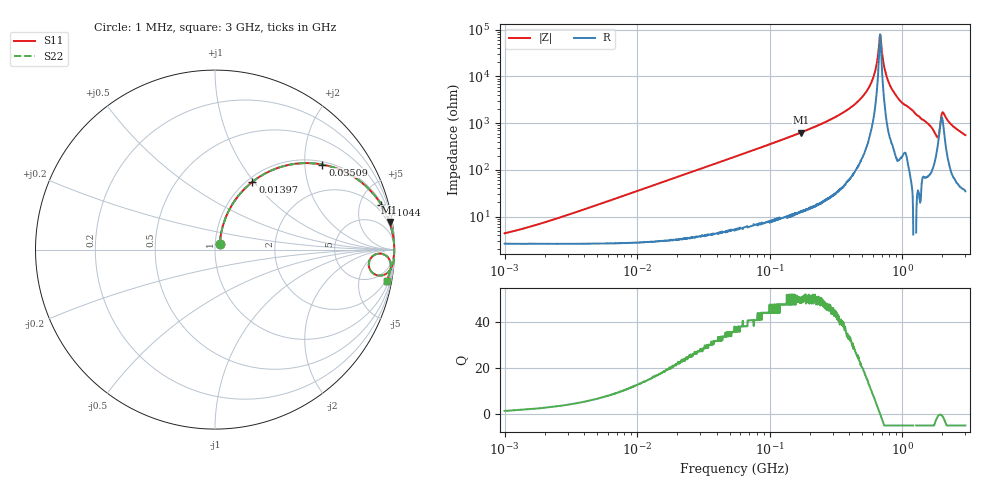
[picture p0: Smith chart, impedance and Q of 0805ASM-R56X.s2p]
!s-Parameter Generated by FASTRON Sdn. Bhd.
!FASTRON P/N : 0805ASM-R56X
!Keysight Technologies: E4991B_MY54100416_A.01.15
!Date: Fri Jun 19 14:53:02 2026
!Version  :Rev00  Fri Jun 19 14:53:02 2026
!Data & Calibration Information:
!Freq  S11  S21  S12  S22
!PortZ  Port1:50+j0  Port2:50+j0
!When reading reference impedance value at option line is always used.
! Remarks : This data is being provided solely for informational purposes.
# Hz S dB R 50
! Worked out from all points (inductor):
!   1601 points, 1 MHz to 3 GHz, reference 50 ohm
!   read as one part in series: L = 560 nH near 2.216 MHz
!   highest Q = 51.2 at 172.3 MHz (marker M1), where L = 581 nH
!   self-resonance near 682.1 MHz
!   S11 on the Smith chart (normalised r, x): 1 MHz: 1.05, +0.07; 13.97 MHz: 1.06, +0.98; 35.09 MHz: 1.08, +2.45; 104.4 MHz: 1.16, +7.37; 3 GHz: 2, -11
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1000000  -27.40 51.3  -0.23 -2.0  -0.23 -2.0  -27.40 51.3
3804036  -17.60 71.5  -0.30 -7.4  -0.30 -7.4  -17.60 71.5
1.397259e7  -7.31 61.1  -1.14 -25.5  -1.14 -25.5  -7.31 61.1
1.447069e7  -7.07 60.4  -1.20 -26.3  -1.20 -26.3  -7.07 60.4
3.508696e7  -2.35 38.4  -4.13 -49.7  -4.13 -49.7  -2.35 38.4
5.504702e7  -1.13 27.1  -6.82 -61.3  -6.82 -61.3  -1.13 27.1
1.044488e8  -0.36 15.1  -11.70 -73.7  -11.70 -73.7  -0.36 15.1
1.722755e8  -0.13 9.0  -16.10 -79.9  -16.10 -79.9  -0.13 9.0
2.083556e8  -0.09 7.2  -18.00 -81.6  -18.00 -81.6  -0.09 7.2
3.649251e8  -0.03 3.3  -24.80 -85.2  -24.80 -85.2  -0.03 3.3
5.077325e8  -0.01 1.5  -31.70 -85.6  -31.70 -85.6  -0.01 1.5
6.049187e8  -0.01 0.6  -39.50 -82.4  -39.50 -82.4  -0.01 0.6
6.787043e8  -0.01 0.0  -57.30 -20.3  -57.30 -20.3  -0.01 0.0
6.993907e8  -0.01 -0.1  -52.10 59.1  -52.10 59.1  -0.01 -0.1
7.38967e8  -0.01 -0.4  -43.00 80.3  -43.00 80.3  -0.01 -0.4
7.925923e8  -0.01 -0.8  -37.40 84.6  -37.40 84.6  -0.01 -0.8
9.730857e8  -0.02 -1.9  -29.40 84.6  -29.40 84.6  -0.02 -1.9
1.800756e9  -0.65 -9.0  -15.50 60.1  -15.50 60.1  -0.65 -9.0
1.86495e9  -1.25 -6.8  -15.20 36.1  -15.20 36.1  -1.25 -6.8
2.050964e9  -0.27 -2.9  -24.60 57.1  -24.60 57.1  -0.27 -2.9
2.383164e9  -0.14 -6.3  -19.20 78.7  -19.20 78.7  -0.14 -6.3
3e9  -0.24 -10.2  -15.10 76.2  -15.10 76.2  -0.24 -10.2
